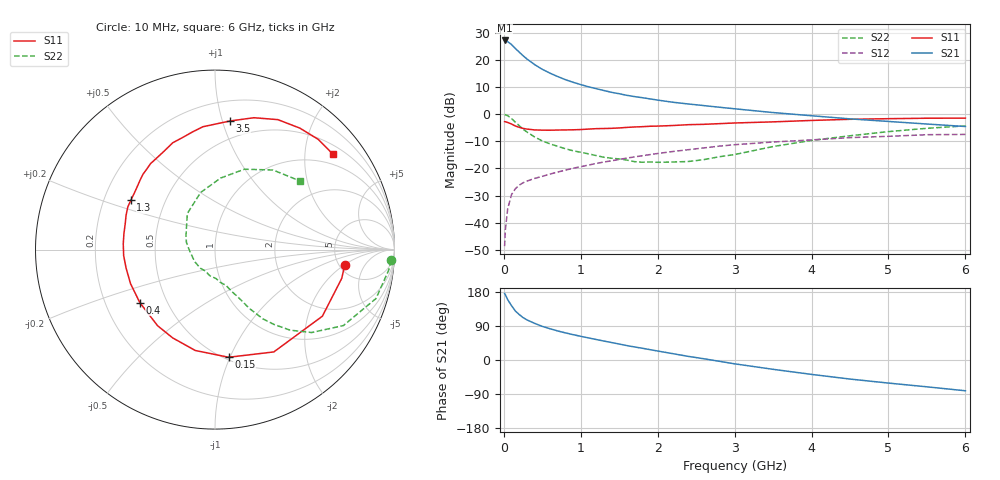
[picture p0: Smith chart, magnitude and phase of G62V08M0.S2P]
! SIEMENS Small Signal Semiconductors
! BFG193
! Si NPN RF Bipolar Junction Transistor in SOT223
! VCE = 2 V  IC = 8 mA
! Common Emitter S-Parameters:  August  1996
# GHz  S  MA  R  50
!  f  S11  S21  S12  S22
! GHz  MAG  ANG  MAG  ANG  MAG  ANG  MAG  ANG
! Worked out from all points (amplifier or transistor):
!   36 points, 10 MHz to 6 GHz, reference 50 ohm
!   highest |S21| = 27.2 dB at 10 MHz (marker M1)
!   |S21| within 3 dB of that: start of sweep to 150.7 MHz
!   unconditionally stable (mu >= 1): 938.9 MHz to 2.697 GHz
!   at 250 MHz: K = 0.47, MSG = 23.4 dB, |S12| = -25.3 dB
!   at 1.4 GHz: K = 1.08, MAG = 10.8 dB, |S12| = -17.2 dB
!   at 6 GHz: K = 0.91, MSG = 1.5 dB, |S12| = -7.5 dB
!   S11 on the Smith chart (normalised r, x): 10 MHz: 5.60, -2.02; 150 MHz: 0.52, -0.99; 400 MHz: 0.35, -0.28; 1.3 GHz: 0.32, +0.25; 3.5 GHz: 0.35, +1.06; 6 GHz: 0.71, +2.66
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0.01  0.728 -6.7  22.78 175.5  0.0037 88.3  0.9834 -3.5
0.02  0.7241 -12.8  22.6 172.2  0.0074 83.4  0.9739 -6.9
0.05  0.704 -31.8  21.64 159.1  0.0181 75.4  0.9375 -16.9
0.1  0.6576 -60.1  19.14 143.4  0.0329 63.9  0.8312 -30.6
0.15  0.6046 -82.8  16.16 129.3  0.0424 55.5  0.71 -40.6
0.2  0.5726 -101.1  13.9 119.9  0.0493 50.8  0.6137 -47.0
0.25  0.5456 -115.6  11.93 111.9  0.0545 47.4  0.5287 -51.9
0.3  0.5313 -127.0  10.39 105.9  0.0585 46.4  0.47 -55.3
0.4  0.5125 -144.8  8.189 96.7  0.0655 44.8  0.3797 -59.7
0.5  0.5075 -158.0  6.695 88.7  0.0715 44.2  0.3214 -62.4
0.6  0.506 -168.2  5.684 82.5  0.0788 44.7  0.284 -64.9
0.7  0.51 -176.3  4.931 76.7  0.0858 44.9  0.2555 -67.8
0.9  0.5152 169.9  3.871 66.9  0.1009 44.8  0.2117 -72.4
1.1  0.531 158.9  3.195 58.3  0.1153 44.3  0.1858 -80.5
1.3  0.5437 149.6  2.727 50.0  0.1314 42.8  0.1608 -88.3
1.6  0.5701 136.9  2.221 38.0  0.1552 39.2  0.1425 -105.3
2.2  0.6178 117.2  1.656 16.6  0.2054 29.9  0.1314 -148.7
2.8  0.6683 100.6  1.342 -3.4  0.2576 18.4  0.1642 165.8
3.5  0.7212 83.4  1.07 -24.6  0.3071 2.4  0.2533 127.5
4.5  0.8043 64.2  0.819 -50.3  0.3696 -17.3  0.3999 85.5
5.5  0.8415 46.9  0.658 -70.8  0.4184 -41.2  0.5488 53.9
6  0.8452 39.0  0.592 -81.2  0.4232 -55.0  0.6082 39.0
